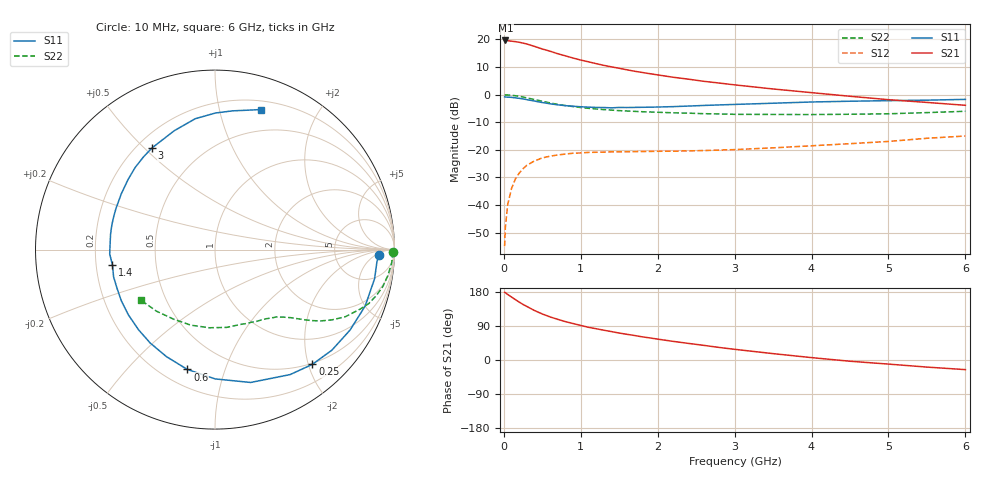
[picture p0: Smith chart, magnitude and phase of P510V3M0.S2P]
! SIEMENS Small Signal Semiconductors
! BFP183
! Si NPN RF Bipolar Junction Transistor in SOT143
! VCE = 10 V  IC = 3 mA
! Common Emitter S-Parameters:  March  1996
# GHz  S  MA  R  50
!  f  S11  S21  S12  S22
! GHz  MAG  ANG  MAG  ANG  MAG  ANG  MAG  ANG
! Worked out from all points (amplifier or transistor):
!   36 points, 10 MHz to 6 GHz, reference 50 ohm
!   highest |S21| = 19.7 dB at 20 MHz (marker M1)
!   |S21| within 3 dB of that: start of sweep to 489.9 MHz
!   unconditionally stable (mu >= 1): 1.979 GHz to 5.845 GHz
!   at 250 MHz: K = 0.15, MSG = 22.7 dB, |S12| = -26.8 dB
!   at 1.4 GHz: K = 0.76, MSG = 15.4 dB, |S12| = -20.7 dB
!   at 6 GHz: K = 0.97, MSG = 5.6 dB, |S12| = -15.0 dB
!   S11 on the Smith chart (normalised r, x): 10 MHz: 19, -7; 250 MHz: 0.48, -2.07; 600 MHz: 0.30, -0.75; 1.4 GHz: 0.27, -0.07; 3 GHz: 0.26, +0.53; 6 GHz: 0.28, +1.35
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0.01  0.9117 -2.0  9.574 178.6  0.0018 83.0  0.9944 -0.8
0.02  0.9047 -4.4  9.606 177.5  0.004 84.4  0.989 -1.7
0.05  0.9039 -10.3  9.523 173.0  0.0102 85.0  0.9877 -4.1
0.15  0.8758 -30.8  9.145 159.3  0.0297 72.2  0.9575 -12.4
0.2  0.8591 -40.7  8.909 152.8  0.038 67.3  0.9347 -15.9
0.25  0.8385 -49.7  8.589 146.5  0.0456 62.8  0.9074 -19.4
0.3  0.8124 -59.0  8.282 141.2  0.0527 58.4  0.874 -22.3
0.4  0.7664 -75.0  7.491 130.4  0.0632 50.8  0.8163 -27.3
0.5  0.7205 -89.9  6.727 121.5  0.0715 44.4  0.7601 -31.0
0.6  0.6853 -103.0  6.144 113.8  0.0768 39.4  0.7105 -34.0
0.7  0.6547 -114.4  5.522 107.3  0.0808 35.3  0.6683 -36.3
0.8  0.6335 -124.7  5.058 101.3  0.084 31.8  0.6353 -38.0
0.9  0.6173 -133.6  4.613 96.2  0.087 29.4  0.6092 -39.4
1.1  0.5947 -151.3  3.944 86.3  0.09 25.2  0.5666 -42.0
1.4  0.5777 -171.5  3.191 74.9  0.092 21.6  0.5254 -45.7
1.8  0.591 166.4  2.525 61.1  0.0935 19.5  0.4912 -50.6
2.2  0.6076 149.2  2.071 49.2  0.0948 19.4  0.4699 -56.4
3  0.6661 121.9  1.506 28.2  0.1012 21.7  0.4408 -70.9
3.5  0.7003 108.9  1.269 16.8  0.1088 23.3  0.4382 -81.5
4.5  0.7611 89.8  0.936 -3.3  0.1295 24.2  0.4419 -107.7
5.5  0.7962 77.2  0.724 -18.7  0.1623 22.6  0.4735 -133.6
6  0.822 71.7  0.642 -25.4  0.1784 19.3  0.5003 -145.9
